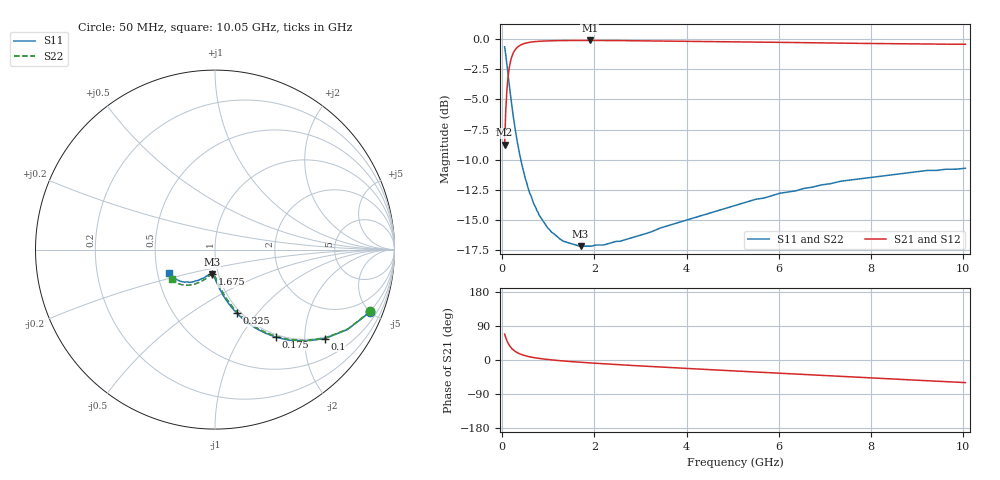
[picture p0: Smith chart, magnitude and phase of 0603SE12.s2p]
! AVX Thin Film Operation		Date: August 2001
! Description: Accu-P® Series, Thin Film, SMD, RF Capacitor
! Part Number: 06035J120FBT
! 50 MHz  -  10.05 GHz
! Serial Measurements
# mhz S db R 50
!	S11		S21		S12		S22
!	dB	Phase	dB	Phase	dB	Phase	dB	Phase
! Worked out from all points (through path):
!   401 points, 50 MHz to 10.05 GHz, reference 50 ohm
!   highest |S21| = -0.09 dB at 1.9 GHz (marker M1); lowest = -8.8 dB at 50 MHz (marker M2)
!   group delay of S21, straight-line fit = 20.3 ps
!   lowest |S11| = -17.2 dB at 1.7 GHz (marker M3), VSWR 1.32, Z = 46.5 - j13 ohm
!   |S11| at or under -10 dB: 400.4 MHz to end of sweep
!   |S22| runs from -17.2 to -0.6 dB; largest |S21 - S12| = 0.00011
!   S11 on the Smith chart (normalised r, x): 50 MHz: 0.96, -4.99; 100 MHz: 0.96, -2.50; 175 MHz: 0.96, -1.44; 325 MHz: 0.96, -0.79; 1.675 GHz: 0.93, -0.26; 10.05 GHz: 0.57, -0.17
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50  -0.62 -21.9  -8.76 68.2  -8.76 68.2  -0.62 -21.7
100  -2.07 -39.0  -4.21 51.1  -4.21 51.1  -2.07 -38.7
125  -2.91 -45.5  -3.11 44.6  -3.11 44.6  -2.91 -45.2
175  -4.54 -55.3  -1.88 34.9  -1.88 34.9  -4.54 -54.8
200  -5.31 -59.0  -1.51 31.2  -1.51 31.2  -5.31 -58.5
250  -6.72 -64.9  -1.04 25.4  -1.04 25.4  -6.72 -64.2
325  -8.52 -71.0  -0.66 19.4  -0.66 19.4  -8.52 -70.1
425  -10.42 -76.5  -0.42 14.0  -0.42 14.0  -10.42 -75.3
550  -12.25 -81.0  -0.27 9.7  -0.27 9.7  -12.25 -79.5
700  -13.79 -84.8  -0.19 6.0  -0.19 6.0  -13.79 -82.9
850  -14.91 -87.5  -0.15 3.4  -0.15 3.4  -14.91 -85.4
1275  -16.66 -93.2  -0.10 -2.0  -0.10 -2.0  -16.66 -90.3
1675  -17.19 -97.2  -0.09 -5.8  -0.09 -5.8  -17.10 -94.0
1700  -17.20 -97.4  -0.09 -6.0  -0.09 -6.0  -17.12 -94.1
1725  -17.20 -97.5  -0.09 -6.2  -0.09 -6.2  -17.15 -94.3
1900  -17.20 -99.0  -0.09 -7.6  -0.09 -7.6  -17.20 -95.7
2600  -16.74 -104.6  -0.10 -12.8  -0.10 -12.8  -16.70 -100.6
3400  -15.73 -109.9  -0.13 -18.4  -0.13 -18.4  -15.72 -105.9
5050  -13.82 -121.4  -0.20 -29.0  -0.20 -29.0  -13.76 -116.4
6725  -12.29 -132.0  -0.28 -39.3  -0.28 -39.3  -12.20 -126.0
8400  -11.29 -143.1  -0.36 -49.6  -0.36 -49.6  -11.19 -136.1
10050  -10.72 -152.8  -0.41 -59.6  -0.41 -59.6  -10.70 -145.6
